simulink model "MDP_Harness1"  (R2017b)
settings: Solver=FixedStepDiscrete  StartTime=0.0  StopTime=2  FixedStep=0.01  RelTol=1e-3  EnableMultiTasking=on
undefined symbols (not defined in the file): sigbuilder_block

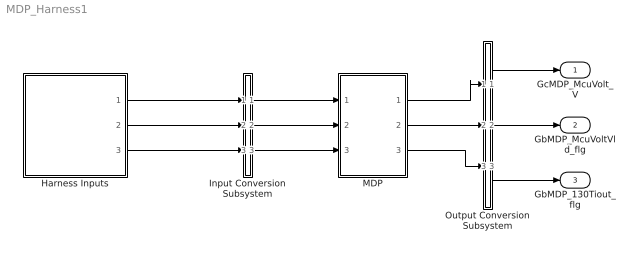
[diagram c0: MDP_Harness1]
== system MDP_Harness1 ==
  Harness Inputs : Subsystem  Tag=STV Subsys  LoadFcn=sigbuilder_block('load');  StartFcn=sigbuilder_block('start');  StopFcn=sigbuilder_block('stop');  ClipboardFcn=sigbuilder_block('clipboard');  mask(Sigbuilder block){tuvar=[0:10]}
      mask init:
      | if ~strcmp(get_param(bdroot(gcb),'SimulationStatus'),'stopped'),tuvar = sigbuilder_block('maskInit'); end
  Input Conversion Subsystem : Subsystem  Tag=__SLT_ICS__  Description=Signal spec. and routing
  MDP : ModelReference  ModelNameDialog=MDP  SimulationMode=Normal  ModelReferenceVersion='M100C100'
  Output Conversion Subsystem : Subsystem  Tag=__SLT_OCS__  Description=Signal spec. and routing
  GcMDP_McuVolt_V : Outport  OutDataTypeStr=single  PortDimensions=[1]
  GbMDP_McuVoltVld_flg : Outport  Port=2  OutDataTypeStr=boolean  PortDimensions=[1]
  GbMDP_130Tiout_flg : Outport  Port=3  OutDataTypeStr=boolean  PortDimensions=[1]
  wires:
  Harness Inputs/1(GcISP_McuVolt_V) -> Input Conversion Subsystem/1(Inport_1)
  Harness Inputs/2(GbISP_130Tiout_flg) -> Input Conversion Subsystem/2(Inport_2)
  Harness Inputs/3(GbVDP_DiagPermit_flg) -> Input Conversion Subsystem/3(Inport_3)
  Output Conversion Subsystem/1(Outport_1) -> GcMDP_McuVolt_V/1
  Output Conversion Subsystem/2(Outport_2) -> GbMDP_McuVoltVld_flg/1
  Output Conversion Subsystem/3(Outport_3) -> GbMDP_130Tiout_flg/1
  Input Conversion Subsystem/1(Outport_1) -> MDP/1
  Input Conversion Subsystem/2(Outport_2) -> MDP/2
  Input Conversion Subsystem/3(Outport_3) -> MDP/3
  MDP/1 -> Output Conversion Subsystem/1(Inport_1)
  MDP/2 -> Output Conversion Subsystem/2(Inport_2)
  MDP/3 -> Output Conversion Subsystem/3(Inport_3)

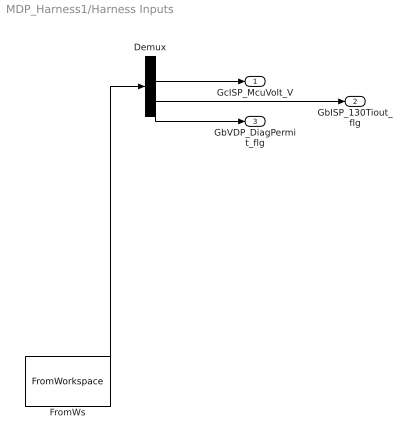
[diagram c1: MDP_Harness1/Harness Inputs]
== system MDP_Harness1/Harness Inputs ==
  Demux : Demux  Tag=STV Demux  Outputs=3
  FromWs : FromWorkspace  Tag=STV FromWs  VariableName=tuvar  SampleTime=0
  GcISP_McuVolt_V : Outport  Tag=STV Outport
  GbISP_130Tiout_flg : Outport  Tag=STV Outport  Port=2
  GbVDP_DiagPermit_flg : Outport  Tag=STV Outport  Port=3
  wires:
  FromWs/1 -> Demux/1
  Demux/1 -> GcISP_McuVolt_V/1
  Demux/2 -> GbISP_130Tiout_flg/1
  Demux/3 -> GbVDP_DiagPermit_flg/1

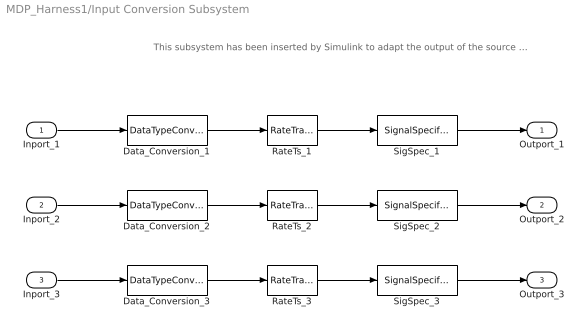
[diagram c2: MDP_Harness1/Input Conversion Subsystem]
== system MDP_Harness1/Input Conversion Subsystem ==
  note: This subsystem has been inserted by Simulink to adapt the output of the source blocks to the interface required by the harnessed component. Modifying the contents of this subsystem may result in compilation and simulation failure.
  Inport_1 : Inport
  Inport_2 : Inport  Port=2
  Inport_3 : Inport  Port=3
  Data_Conversion_1 : DataTypeConversion  OutDataTypeStr=uint16
  Data_Conversion_2 : DataTypeConversion  OutDataTypeStr=boolean
  Data_Conversion_3 : DataTypeConversion  OutDataTypeStr=boolean
  RateTs_1 : RateTransition  OutPortSampleTime=0.01
  RateTs_2 : RateTransition  OutPortSampleTime=0.01
  RateTs_3 : RateTransition  OutPortSampleTime=0.01
  SigSpec_1 : SignalSpecification  OutDataTypeStr=uint16  Unit=V  Dimensions=[1]  SampleTime=0.01
  SigSpec_2 : SignalSpecification  OutDataTypeStr=boolean  Unit=flag  Dimensions=[1]  SampleTime=0.01
  SigSpec_3 : SignalSpecification  OutDataTypeStr=boolean  Unit=flg  Dimensions=[1]  SampleTime=0.01
  Outport_1 : Outport
  Outport_2 : Outport  Port=2
  Outport_3 : Outport  Port=3
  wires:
  SigSpec_1/1 -> Outport_1/1
  RateTs_1/1 -> SigSpec_1/1
  Data_Conversion_1/1 -> RateTs_1/1
  Inport_1/1 -> Data_Conversion_1/1
  SigSpec_2/1 -> Outport_2/1
  RateTs_2/1 -> SigSpec_2/1
  Data_Conversion_2/1 -> RateTs_2/1
  Inport_2/1 -> Data_Conversion_2/1
  SigSpec_3/1 -> Outport_3/1
  RateTs_3/1 -> SigSpec_3/1
  Data_Conversion_3/1 -> RateTs_3/1
  Inport_3/1 -> Data_Conversion_3/1

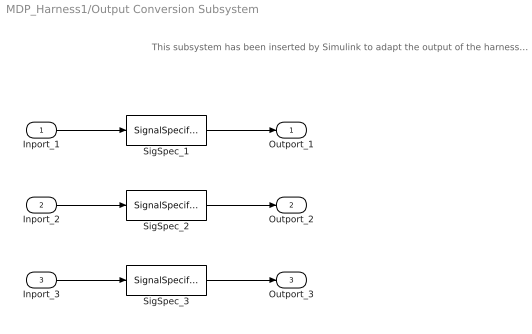
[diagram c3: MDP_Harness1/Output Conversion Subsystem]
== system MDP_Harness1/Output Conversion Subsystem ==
  note: This subsystem has been inserted by Simulink to adapt the output of the harnessed component to the interface required by the sink blocks. Modifying the contents of this subsystem may result in compilation and simulation failure.
  Inport_1 : Inport
  Inport_2 : Inport  Port=2
  Inport_3 : Inport  Port=3
  SigSpec_1 : SignalSpecification  OutDataTypeStr=single  Unit=V  Dimensions=[1]  SampleTime=0.01
  SigSpec_2 : SignalSpecification  OutDataTypeStr=boolean  Unit=flg  Dimensions=[1]  SampleTime=0.01
  SigSpec_3 : SignalSpecification  OutDataTypeStr=boolean  Unit=flg  Dimensions=[1]  SampleTime=0.01
  Outport_1 : Outport
  Outport_2 : Outport  Port=2
  Outport_3 : Outport  Port=3
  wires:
  Inport_1/1 -> SigSpec_1/1
  SigSpec_1/1 -> Outport_1/1
  Inport_2/1 -> SigSpec_2/1
  SigSpec_2/1 -> Outport_2/1
  Inport_3/1 -> SigSpec_3/1
  SigSpec_3/1 -> Outport_3/1
